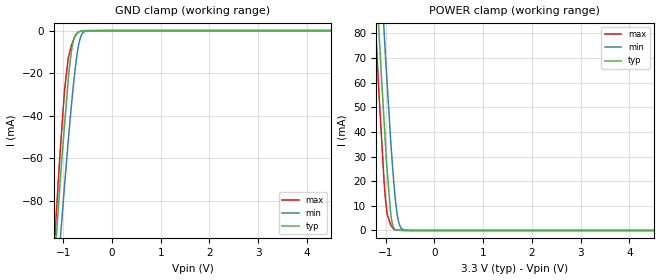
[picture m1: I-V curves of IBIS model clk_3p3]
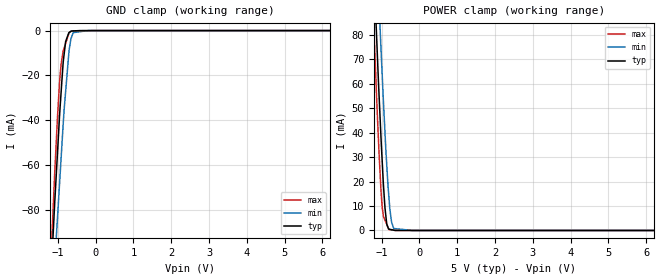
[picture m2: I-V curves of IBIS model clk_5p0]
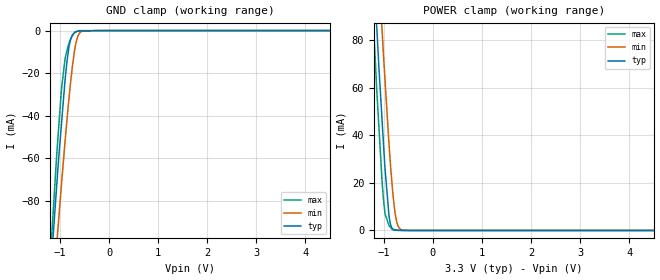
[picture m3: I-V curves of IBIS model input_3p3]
|Texas Instruments Incorporated
|12 Bit, 8 MSPS ADC with Dual Ch., DSP/uP Interface, 16X FIFO, Channel Autoscan,
|Low Power
| Marketing part#   Digital Voltage Range   Package-type   #pins
| THS12082CDA   3.0V - 5.25V   TSSOP   32
| THS12082CDAG4   3.0V - 5.25V   TSSOP   32
| THS12082CDAR   3.0V - 5.25V   TSSOP   32
| THS12082CDARG4   3.0V - 5.25V   TSSOP   32
| THS12082IDA   3.0V - 5.25V   TSSOP   32
| THS12082IDAG4   3.0V - 5.25V   TSSOP   32
| THS12082IDAR   3.0V - 5.25V   TSSOP   32
| THS12082IDARG4   3.0V - 5.25V   TSSOP   32
[IBIS Ver]   3.2
[File name]   ths12082.ibs
|SIMDE Ver   V3.0 - 201101 - Build 457
[File Rev]   1.0
[Date]   12/21/2011
[Source]
| Texas Instruments Incorporated.
| Analog-eLab Design Center, HPA
| 12500 TI Blvd
| Dallas, TX -75243
| e-mail: elab_scm_ibis@list.ti.com
[Notes]   Revision History:
| Rev 1.0: 12/21/2011
| - Initial version of the model
| - Model generated from simulations in TISPICE
| - Model matched to SPICE simulation
| - C_comp although listed in numerical order of value are
|   obtained from varying PVT conditions. For PVT conditions for
|   each specific value refer the buffer description under
|   respective [Model]. IBIS model user is responsible for using
|   appropriate C_comp to simulate for Signal Integrity.
| - Model names with a trailing _3p3 contains the model for
|   3.3V [3.0V and 3.6V]. Model names with a trailing _5 contains
|   the model for 5.0V [4.75V and 5.25V].
[Disclaimer]
| This model is designed as an aid for customers of Texas Instruments.
| TI and its licensors and suppliers make no warranties, either expressed
| or implied, with respect to this  model, including the warranties of
| merchantability or fitness for a particular purpose. The model is
| provided solely on an "as is" basis. The entire risk as to its quality
| and performance is with the customer.
[Copyright]
 (C) Copyright 2011 Texas Instruments Incorporated.All rights reserved.
|   THS12082
[Component]   THS12082
[Manufacturer]   TI
[Package]   |32 TSSOP   -  DA package
|   typ   min   max
R_pkg   0.22349   0.20935   0.24230
L_pkg   3.56109nH   2.82748nH   5.26107nH
C_pkg   0.76313pF   0.65107pF   0.89665pF
[Pin]  signal_name   model_name   R_pin   L_pin   C_pin
1   D0   DB   0.23660   5.10197nH  0.88632pF
2   D1   DB   0.22824   4.15037nH  0.83153pF
3   D2   DB   0.23170   3.54048nH  0.76928pF
4   D3   DB   0.22790   3.45427nH  0.76690pF
5   D4   DB   0.21901   3.21370nH  0.75682pF
6   D5   DB   0.21584   3.07611nH  0.69847pF
7   BVDD   POWER   0.21269   2.91205nH  0.67046pF
8   BGND   GND   0.21047   2.79716nH  0.64638pF
9   D6   DB   0.21377   2.82748nH  0.66907pF
10   D7   DB   0.21458   2.92175nH  0.66849pF
11   D8   DB   0.21614   3.07364nH  0.69753pF
12   D9   DB   0.22067   3.23034nH  0.75697pF
13   RA0/D10   DB   0.22630   3.43331nH  0.76788pF
14   RA1/D11   DB   0.23221   3.54819nH  0.76968pF
15   CONV_CLK(_CONVST)   CLK   0.22890   4.15953nH  0.83396pF
16   DATA_AV   DATA   0.23697   5.10236nH  0.88787pF
17   DGND   GND   0.23354   5.07864nH  0.88757pF
18   DVDD   POWER   0.22775   4.14883nH  0.83532pF
19   _RD   INPUT   0.22349   3.47204nH  0.77751pF
20   _WR(R/_W)   INPUT   0.21833   3.37323nH  0.76759pF
21   CS1   INPUT   0.21330   3.16831nH  0.75570pF
22   _CS0   INPUT   0.21263   3.05054nH  0.69695pF
23   AVDD   POWER   0.21439   2.92741nH  0.66643pF
24   AGND   GND   0.12364   2.47453nH  0.68936pF
25   REFM   TERM   0.21568   2.83733nH  0.65107pF
26   REFP   TERM   0.21574   2.93112nH  0.67527pF
27   REFOUT   TERM   0.22130   3.11874nH  0.70174pF
28   REFIN   TERM   0.20935   3.13455nH  0.74859pF
29   AINM   TERM   0.21905   3.38287nH  0.72574pF
30   AINP   TERM   0.24112   3.66662nH  0.81322pF
31   _RESET   RST   0.22953   4.35847nH  0.87055pF
32   OV_FL   OVFL   0.24230   5.26107nH  0.89665pF
1000   thermal_pad   NC   0.00004   0.00163nH  3.26032pF
|   Model Selectors
[Model Selector] CLK
clk_3p3  3.3V digital input
clk_5p0  5.0V digital input
[Model Selector] INPUT
input_3p3  3.3V digital input
input_5p0  5.0V digital input
[Model Selector] RST
rst_3p3  3.3V digital input
rst_5p0  5.0V digital input
[Model Selector] OVFL
ovfl_3p3  3.3V digital output
ovfl_5p0  5.0V digital output
[Model Selector] DATA
data_3p3  3.3V digital output
data_5p0  5.0V digital output
[Model Selector] DB
db_3p3  3.3V digital I/O
db_5p0  5.0V digital I/O
[Model Selector] TERM
term_3-3V  3.3V nominal termination
term_5-0V  5.0V nominal termination
[Model] term_3-3V
Model_type Terminator
C_comp   1.0e-20F  1.0e-20F  1.0e-20F
|   typ   min   max
[Voltage Range]   3.3V   3.0V   3.6V
[POWER Clamp Reference]   3.3V   3.0V   3.6V
[GND Clamp Reference]   0V   0V   0V
|Ambient Temperature   25   125   -55
|Junction Temperature
[Temperature Range]   27   125   -55
[Model] term_5-0V
Model_type Terminator
C_comp   1.0e-20F  1.0e-20F  1.0e-20F
|   typ   min   max
[Voltage Range]   5.0V   4.75V   5.25V
[POWER Clamp Reference]   5.0V   4.75V   5.25V
[GND Clamp Reference]   0V   0V   0V
|Ambient Temperature   25   125   -55
|Junction Temperature
[Temperature Range]   27   125   -55
| Models and submodels in the file (14): clk_3p3 (Input), clk_5p0 (Input), input_3p3 (Input), input_5p0 (Input), rst_3p3 (Input), rst_5p0 (Input), ovfl_3p3 (Output), ovfl_5p0 (Output), data_3p3 (Output), data_5p0 (Output), db_3p3 (I/O), db_5p0 (I/O), term_3-3V (Terminator), term_5-0V (Terminator)
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|   clk_3p3 Model
[Model]   clk_3p3
Model_type   Input
Vinl = 0.6
Vinh = 2
|   typ   min   max
|   (nom PVT)   (fast PVT)   (slow PVT)
C_comp   1.052e-12   1.043e-12   1.060e-12
| Where nom  PVT is Nominal Process, 3.3V, 27C
|   Fast PVT is Strong Process,  3.6V, -55C
|   Slow PVT is Weak Process,   3V, 125C
[Voltage Range]   3.3   3   3.6
|Ambient Temperature   25   125   -55
|Junction Temperature
[Temperature Range]   27   125   -55
[Power Clamp Reference]   3.3   3   3.6
[GND Clamp Reference]   0   0   0
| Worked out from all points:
|   GND clamp passes 1 mA (typ) near -0.71 V on its own axis
|   POWER clamp passes 1 mA (typ) near -0.83 V on its own axis
[GND Clamp]
|   Voltage   I(typ)   I(min)   I(max)
-3.3V     -935.6mA   -897.7mA   -1.009A
-1.224V   -123.9mA   -149mA     -116.7mA
-1.084V   -77.72mA   -105.2mA   -63.84mA
-1.036V   -62.17mA   -91.12mA   -48mA
-972mV    -44.01mA   -72.35mA   -27.55mA
-896.4mV  -22.7mA    -51.46mA   -12.8mA
-858mV    -14.18mA   -41.44mA   -9.297mA
-792mV    -4.695mA   -25.64mA   -4.36mA
-696.3mV  -754.6uA   -8.26mA    -763.9uA
-591mV    -157.8uA   -849.9uA   -43.98uA
-285mV    -75.61uA   -318nA     -32.66nA
6.6V      0A         0A         0A
[POWER Clamp]
|   Voltage   I(typ)   I(min)   I(max)
-3.3V     973mA      989.7mA    970.3mA
-1.29V    137.6mA    174.6mA    114.3mA
-1.158V   87.39mA    124.9mA    62.68mA
-1.141V   81.22mA    118.9mA    56.13mA
-1.037V   45.16mA    81.65mA    20.52mA
-975.6mV  25.23mA    61mA       6.972mA
-897.6mV  6.664mA    36.03mA    2.234mA
-813.6mV  555.7uA    14.8mA     241.2uA
-765mV    191.6uA    6.477mA    181.2uA
-714mV    56.08uA    2.037mA    118.2uA
-591mV    10.98uA    69.36uA    14.83uA
6.6V      0A         0A         0A
|   clk_5p0 Model
[Model]   clk_5p0
Model_type   Input
Vinl = 0.6
Vinh = 2.6
|   typ   min   max
|   (nom PVT)   (fast PVT)   (slow PVT)
C_comp   9.597e-13   9.523e-13   9.672e-13
| Where nom  PVT is Nominal Process, 5V, 27C
|   Fast PVT is Strong Process,  5.25V, -55C
|   Slow PVT is Weak Process,   4.75V, 125C
[Voltage Range]   5   4.75   5.25
|Ambient Temperature   25   125   -55
|Junction Temperature
[Temperature Range]   27   125   -55
[Power Clamp Reference]   5   4.75   5.25
[GND Clamp Reference]   0   0   0
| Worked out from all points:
|   GND clamp passes 1 mA (typ) near -0.71 V on its own axis
|   POWER clamp passes 1 mA (typ) near -0.83 V on its own axis
[GND Clamp]
|   Voltage   I(typ)   I(min)   I(max)
-5V       -1.642A    -1.561A    -1.765A
-1.306V   -152.3mA   -174.9mA   -149mA
-1.088V   -78.49mA   -106.4mA   -65.35mA
-1.036V   -62.48mA   -90.78mA   -47.43mA
-945mV    -35.31mA   -65.66mA   -20.86mA
-855mV    -13.59mA   -40.68mA   -8.966mA
-795mV    -4.964mA   -27.44mA   -5.832mA
-707.7mV  -970.8uA   -9.742mA   -1.275mA
-640.5mV  -218.9uA   -3.11mA    -155.4uA
-593.8mV  -169.5uA   -909.9uA   -144.1uA
-190mV    0A         -23.35nA   -46.1uA
10V       0A         0A         0A
[POWER Clamp]
|   Voltage   I(typ)   I(min)   I(max)
-5V       1.711A     1.714A     1.716A
-1.306V   144.9mA    181.1mA    122.6mA
-1.118V   74.11mA    111mA      49.44mA
-1.05V    49.52mA    86.13mA    26.27mA
-981.8mV  27.66mA    62.87mA    9.228mA
-910mV    9.161mA    39.94mA    4.226mA
-860mV    2.43mA     25.95mA    2.402mA
-803.3mV  525.6uA    13.03mA    330.8uA
-736.2mV  316.1uA    3.495mA    205.4uA
-679.3mV  137.9uA    817.9uA    98.62uA
-190mV    0A         0A         7.728uA
10V       0A         0A         0A
|   input_3p3 Model
[Model]   input_3p3
Model_type   Input
Vinl = 0.6
Vinh = 2
|   typ   min   max
|   (nom PVT)   (fast PVT)   (slow PVT)
C_comp   1.052e-12   1.043e-12   1.060e-12
| Where nom  PVT is Nominal Process, 3.3V, 27C
|   Fast PVT is Strong Process,  3.6V, -55C
|   Slow PVT is Weak Process,   3V, 125C
[Voltage Range]   3.3   3   3.6
|Ambient Temperature   25   125   -55
|Junction Temperature
[Temperature Range]   27   125   -55
[Power Clamp Reference]   3.3   3   3.6
[GND Clamp Reference]   0   0   0
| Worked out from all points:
|   GND clamp passes 1 mA (typ) near -0.71 V on its own axis
|   POWER clamp passes 1 mA (typ) near -0.83 V on its own axis
[GND Clamp]
|   Voltage   I(typ)   I(min)   I(max)
-3.3V     -935.6mA   -897.7mA   -1.009A
-1.224V   -123.9mA   -149mA     -116.7mA
-1.084V   -77.72mA   -105.2mA   -63.84mA
-1.036V   -62.17mA   -91.12mA   -48mA
-972mV    -44.01mA   -72.35mA   -27.55mA
-896.4mV  -22.7mA    -51.46mA   -12.8mA
-858mV    -14.18mA   -41.44mA   -9.297mA
-792mV    -4.695mA   -25.64mA   -4.36mA
-696.3mV  -754.6uA   -8.26mA    -763.9uA
-591mV    -157.8uA   -849.9uA   -43.98uA
-285mV    -75.61uA   -318nA     -32.66nA
6.6V      0A         0A         0A
[POWER Clamp]
|   Voltage   I(typ)   I(min)   I(max)
-3.3V     1.011A     1.029A     1.007A
-1.284V   140.1mA    178.7mA    115.5mA
-1.158V   90.48mA    129.5mA    64.64mA
-1.141V   84.07mA    123.3mA    57.84mA
-1.033V   45.33mA    83.19mA    19.86mA
-975.6mV  25.92mA    63.06mA    7.004mA
-897.6mV  6.761mA    37.1mA     2.234mA
-813.6mV  556.5uA    15.12mA    241.2uA
-765mV    191.7uA    6.561mA    181.2uA
-714mV    57.93uA    2.047mA    118.2uA
-591mV    10.98uA    69.38uA    14.83uA
6.6V      0A         0A         0A
